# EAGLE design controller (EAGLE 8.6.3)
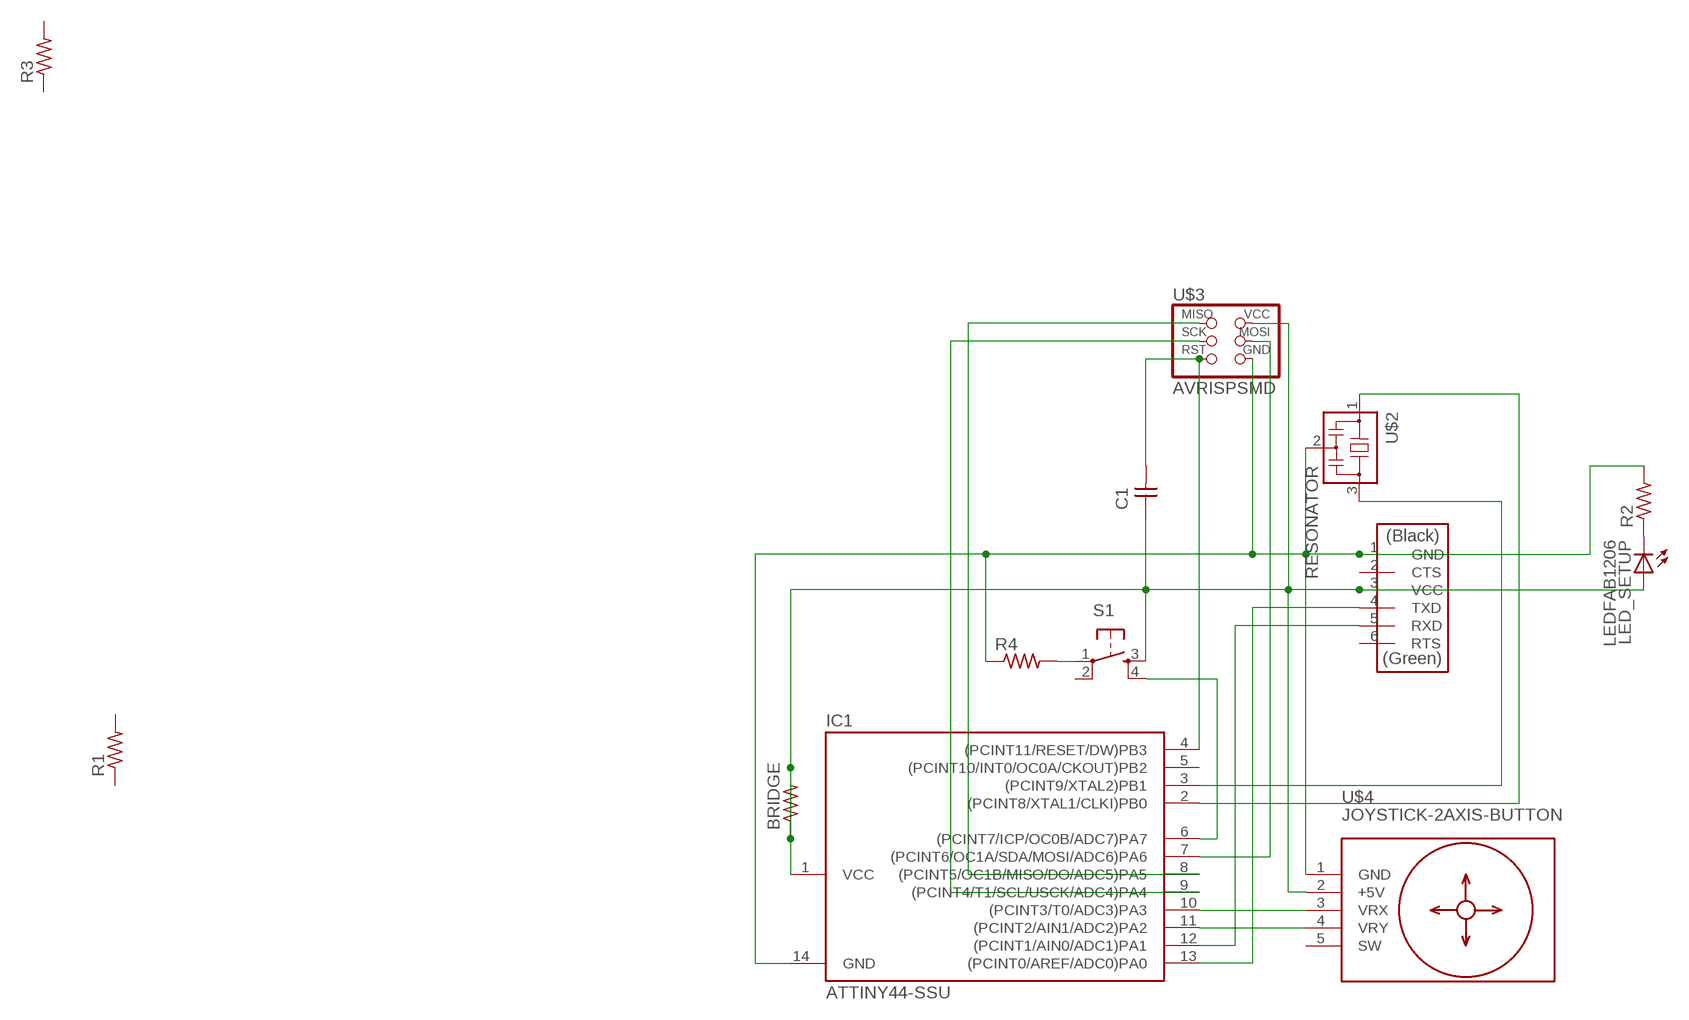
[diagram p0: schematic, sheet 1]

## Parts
BRIDGE  RES-US1206FAB  [R1206FAB]
C1  CAP-UNPOLARIZEDFAB  [C1206FAB]
IC1  ATTINY44-SSU  [SOIC14]
LED_SETUP  LEDFAB1206  [LED1206FAB]
R1  RES-US1206FAB  [R1206FAB]
R2  RES-US1206FAB  [R1206FAB]
R3  RES-US1206FAB  [R1206FAB]
R4  RES-US1206FAB  [R1206FAB]
S1  6MM_SWITCH6MM_SWITCH  [6MM_SWITCH]
U$1  FTDI-SMD-HEADER  [1X06SMD]
U$2  RESONATOR  [EFOBM]
U$3  AVRISPSMD  [2X03SMD]
U$4  JOYSTICK-2AXIS-BUTTON  [JOYSTICK-2AXIS-BUTTON]

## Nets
GND: IC1.14(GND) R2.2 R4.1 U$1.1(GND) U$2.2 U$3.6(GND) U$4.1(GND)
N$1: IC1.11((PCINT2/AIN1/ADC2)PA2) U$4.4(VRY)
N$2: IC1.10((PCINT3/T0/ADC3)PA3) U$4.3(VRX)
N$3: R4.2 S1.1(P)
N$4: IC1.6((PCINT7/ICP/OC0B/ADC7)PA7) S1.4(S1)
N$5: LED_SETUP.2(C) R2.1
N$6: IC1.2((PCINT8/XTAL1/CLKI)PB0) U$2.1
N$7: IC1.13((PCINT0/AREF/ADC0)PA0) U$1.4(TXD)
N$8: IC1.12((PCINT1/AIN0/ADC1)PA1) U$1.5(RXD)
N$9: IC1.3((PCINT9/XTAL2)PB1) U$2.3
N$10: C1.2 IC1.4((PCINT11/RESET/DW)PB3) U$3.5(RST)
N$14: IC1.9((PCINT4/T1/SCL/USCK/ADC4)PA4) U$3.3(SCK)
N$15: IC1.8((PCINT5/OC1B/MISO/DO/ADC5)PA5) U$3.1(MISO)
N$16: IC1.7((PCINT6/OC1A/SDA/MOSI/ADC6)PA6) U$3.4(MOSI)
VCC: BRIDGE.1 BRIDGE.2 C1.1 IC1.1(VCC) LED_SETUP.1(A) S1.3(S) U$1.3(VCC) U$3.2(VCC) U$4.2(+5V)
Unconnected: IC1.5((PCINT10/INT0/OC0A/CKOUT)PB2) R1.1 R1.2 R3.1 R3.2 S1.2(P1) U$1.2(CTS) U$1.6(RTS) U$4.5(SW)

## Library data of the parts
BRIDGE R1-R4 = fab:RES-US: Resistor (US Symbol)
C1 = fab:CAP-UNPOLARIZED
IC1 = fab:ATTINY44
LED_SETUP = fab:LED: LED
S1 = fab:6MM_SWITCH: OMRON SWITCH
U$1 = fab:FTDI-SMD-HEADER
U$2 = fab:RESONATOR
U$3 = fab:AVRISP
U$4 = diy-modules:JOYSTICK-2AXIS-BUTTON: 2-Axis Analog Joystick with Push Button Tutorial is available here: http://henrysbench.capnfatz.com/henrys-bench/arduino-sensors-and-input/arduino-ps2-joystick-tutorial-keyes-ky-023-deek-robot/ Click here to find device on ebay.com

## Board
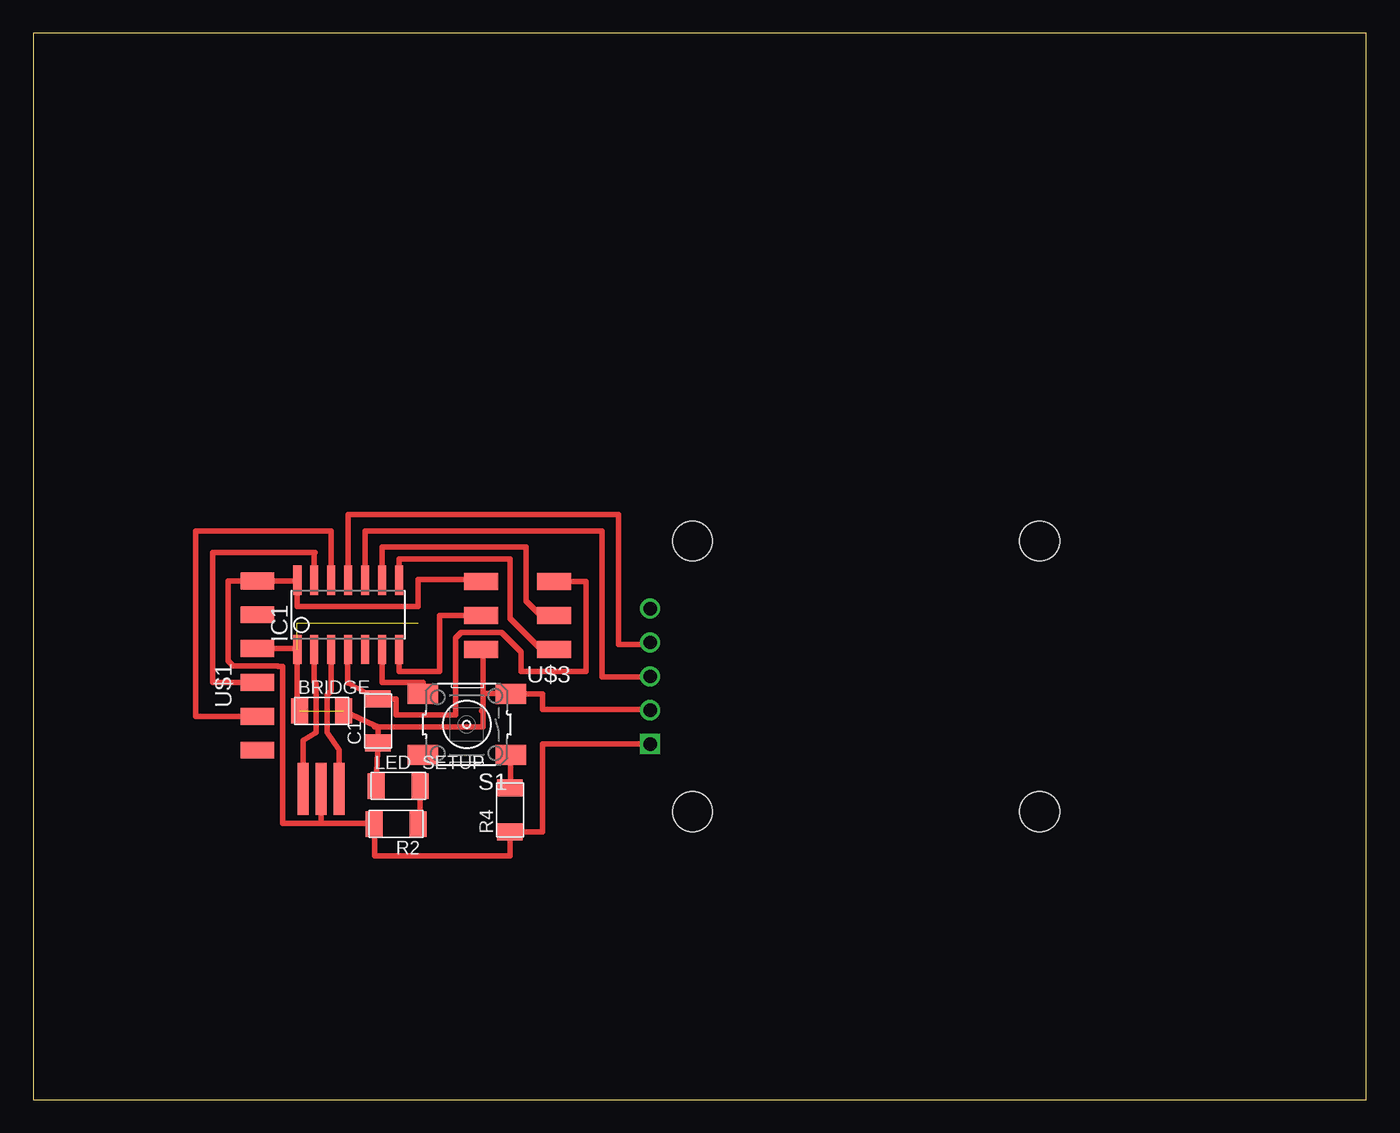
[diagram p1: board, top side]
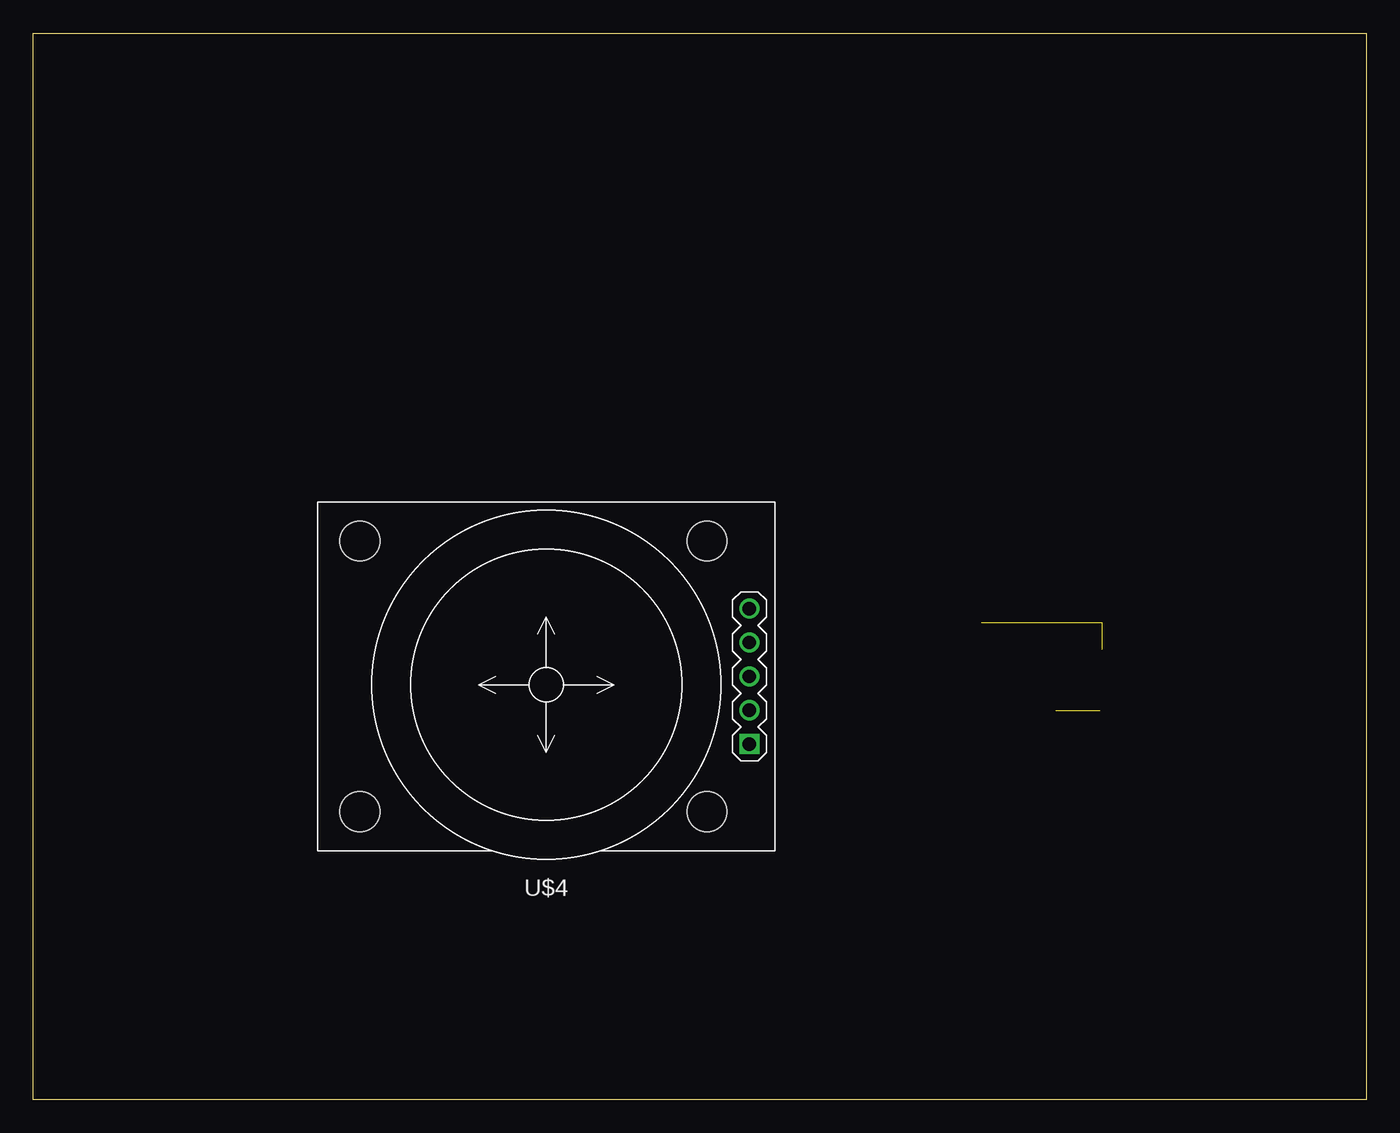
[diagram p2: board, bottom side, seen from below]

Size 100 x 80 mm. Coordinates in mm from the lower left corner, seen from the top.
Outline: 0,0 100,0 100,80 0,80 0,0
Copper layers (1*16): Top 0.035mm / dielectric 1.5mm / Bottom 0.035mm
Design rules "default *": minimum track width 6mil, minimum drill 0.35mm, track to track 16mil, track to pad 16mil, pad to pad 16mil, via to via 16mil, smd to smd 16mil, copper to edge 40mil, drill to drill 6mil, minimum pad ring 10mil, minimum via ring 8mil, stop-mask expansion 4mil, vias tented up to drill 0mil, thermal gap 10mil

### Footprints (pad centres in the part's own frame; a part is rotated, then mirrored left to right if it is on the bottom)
R1206FAB = smd 1.27 x 1.905: 1 -1.651,0; 2 1.651,0
C1206FAB = smd 1.27 x 1.905: 1 -1.651,0; 2 1.651,0
SOIC14 = smd 0.61 x 2.21: 1 -3.81,-2.603; 2 -2.54,-2.603; 3 -1.27,-2.603; 4 0,-2.603; 5 1.27,-2.603; 6 2.54,-2.603; 7 3.81,-2.603; 8 3.81,2.603; 9 2.54,2.603; 10 1.27,2.603; 11 0,2.603; 12 -1.27,2.603; 13 -2.54,2.603; 14 -3.81,2.603
LED1206FAB = smd 1.27 x 1.905: 1 -1.651,0; 2 1.651,0
6MM_SWITCH = smd 2.286 x 1.524: 1 -3.302,2.286; 2 3.302,2.286; 3 -3.302,-2.286; 4 3.302,-2.286
1X06SMD = smd 2.54 x 1.27: 1 0,6.35; 2 0,3.81; 3 0,1.27; 4 0,-1.27; 5 0,-3.81; 6 0,-6.35
EFOBM = smd 0.8 x 3.9: 1 -1.35,0; 2 0,0; 3 1.35,0
2X03SMD = smd 2.54 x 1.27: 1 -2.54,2.54; 2 2.92,2.54; 3 -2.54,0; 4 2.92,0; 5 -2.54,-2.54; 6 2.92,-2.54
JOYSTICK-2AXIS-BUTTON = drill 1 square: 1 -15.24,5.08 | drill 1: 2 -15.24,2.54; 3 -15.24,0; 4 -15.24,-2.54; 5 -15.24,-5.08 | hole 3: -12.065,10.16; -12.065,-10.16; 13.97,-10.16; 13.97,10.16

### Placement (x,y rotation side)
BRIDGE  21.64,29.16 0 top
C1  25.86,28.4 90 top
IC1  23.62,36.37 0 top
LED_SETUP  27.38,23.52 0 top
R1  not placed on the board
R2  27.23,20.68 180 top
R3  not placed on the board
R4  35.76,21.74 90 top
S1  32.51,28.14 180 top
U$1  16.81,32.56 0 top
U$2  21.59,23.32 0 top
U$3  36.53,36.32 180 top
U$4  61.52,31.75 180 bottom

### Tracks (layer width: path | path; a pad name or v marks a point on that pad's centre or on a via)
GND
  Top 0.406: U$3.6 33.6,39.01 28.85,39.01 28.85,36.98 19.81,36.98 IC1.14 19.81,38.91 U$1.1 14.63,38.91 14.63,32.92 15.01,32.54 18.34,32.54 18.36,32.51 18.69,32.51 18.69,20.73 21.54,20.73 | 21.54,20.73 21.59,20.78 U$2.2 | 21.54,20.73 25.58,20.73 R2.2 25.6,20.68 25.6,18.29 35.76,18.29 R4.1 38.2,20.09 38.2,26.67 U$4.1
N$1
  Top 0.406: IC1.11 23.62,43.89 43.89,43.89 43.89,34.14 46.69,34.14 U$4.4
N$2
  Top 0.406: IC1.10 24.89,42.67 42.67,42.67 42.67,31.7 46.28,31.7 U$4.3
N$3
  Top 0.406: R4.2 35.81,23.39 S1.1
N$4
  Top 0.406: IC1.6 26.16,31.29 29.26,31.29 29.26,30.43 S1.4
N$5
  Top 0.406: LED_SETUP.2 29.03,20.68 R2.1
N$6
  Top 0.406: IC1.2 21.08,31.34 21.23,31.19 21.23,27.55 20.24,26.96 U$2.1
N$7
  Top 0.406: U$1.4 13.46,31.29 13.46,41.05 21.08,41.05 | IC1.13 21.08,41.05 | 21.08,41.05 21.13,41.05
N$8
  Top 0.406: IC1.12 22.35,42.67 12.19,42.67 12.19,28.75 U$1.5
N$9
  Top 0.406: IC1.3 22.35,30.67 22.05,30.36 22.05,27.53 22.94,26.23 U$2.3
N$10
  Top 0.406: U$3.5 41.45,38.86 41.45,32.11 36.58,32.11 36.58,33.58 35.13,35.03 32.08,35.03 31.7,34.64 31.7,28.85 27.23,28.85 27.23,30.05 C1.2 23.6,31.27 23.57,31.29 23.57,33.77 IC1.4
N$14
  Top 0.406: IC1.9 26.16,41.45 36.98,41.45 36.98,37.39 38.05,36.32 U$3.3
N$15
  Top 0.406: IC1.8 27.43,40.54 35.76,40.54 35.76,36.1 38.08,33.78 U$3.1
N$16
  Top 0.406: IC1.7 27.43,32.11 30.48,32.11 30.48,36.32 U$3.4
VCC  (3 unrouted)
  Top 0.406: U$1.3 19.81,33.83 IC1.1 | IC1.1 19.91,33.77 | U$3.2 33.73,33.78 33.73,30.48 | 33.73,29.26 33.73,30.48 | IC1.1 19.81,29.34 BRIDGE.1 | 33.63,29.16 33.73,29.26 | BRIDGE.2 25.61,28.06 | 25.61,28.06 25.86,27.94 C1.1 25.73,23.9 LED_SETUP.1 | 33.73,29.26 33.73,27.96 25.61,27.96 25.61,28.06 | 33.73,30.48 35.81,30.48 S1.3 38.2,30.43 38.2,29.26 45.47,29.26 U$4.2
